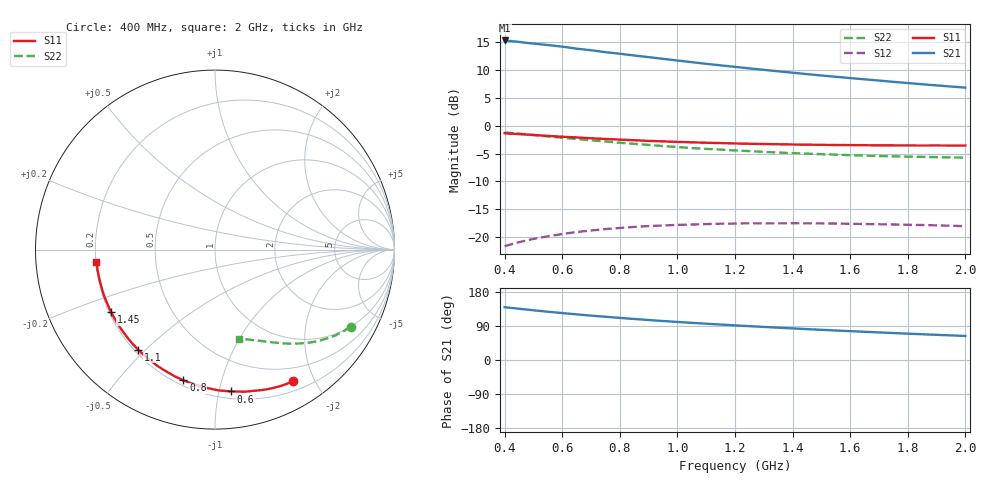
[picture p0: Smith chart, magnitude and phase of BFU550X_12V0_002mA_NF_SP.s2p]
! Filename:  P:\Prog\Test\Noise\ATS_data\Testdata_Net\BFU550X no attenuator noise\BFU550X_APG2013_44_C05_12p0V_002mA_NF_CM01_D.sf
! Date/Time: Fri 26/Jul/2013 14:37:13
! BFU550X_APG2013_44_C05_12p0V_1to10mA_NF_CM01_Bias2_R.sf
! Noise Parameter Data File
! BFU550X_APG2013_44_C05_12p0V_1to10mA_NF_CM01
! Date/time: Thu Jul 25 09:36:35 2013
! VAR V_out= 12.001000
! VAR I_out= 1.995000
! VAR V_in= 0.785500
! VAR I_in= 0.017300
! Device data file deembeded for feedlines and parallel
! Original file: \BFU550X no attenuator noise\BFU550X_APG2013_44_C05_12p0V_002mA_NF_CM01_R.sf
! Feed-files: PR005V01_100713_Feed1.s2p, PR005V01_100713_Feed2.s2p
! Parallel-file: PR005V01_100713_Par.s2p
# MHz S MA R 50
!  Freq-MHz  S11-mag  S11-arg  S21-mag  S21-arg  S12-mag  S12-arg  S22-mag  S22-arg
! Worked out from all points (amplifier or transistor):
!   37 points, 400 MHz to 2 GHz, reference 50 ohm
!   highest |S21| = 15.3 dB at 400 MHz (marker M1)
!   |S21| within 3 dB of that: start of sweep to 902 MHz
!   unconditionally stable (mu >= 1): nowhere
!   at 500 MHz: K = 0.16, MSG = 17.5 dB, |S12| = -20.3 dB
!   at 1.1 GHz: K = 0.33, MSG = 14.4 dB, |S12| = -17.6 dB
!   at 2 GHz: K = 0.62, MSG = 12.4 dB, |S12| = -18.0 dB
!   lowest NFmin = 0.58 dB at 433 MHz
!   S11 on the Smith chart (normalised r, x): 400 MHz: 0.31, -1.71; 600 MHz: 0.25, -1.09; 800 MHz: 0.23, -0.76; 1.1 GHz: 0.22, -0.47; 1.45 GHz: 0.21, -0.27; 2 GHz: 0.20, -0.05
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400  0.8546 -59.3  5.791 139.4  0.08331 55.5  0.8707 -29.8
440  0.8428 -64.5  5.663 136.1  0.08909 52.9  0.8521 -32.0
480  0.8312 -69.3  5.494 132.9  0.09423 50.2  0.8319 -34.2
500  0.824 -71.9  5.434 131.3  0.09676 48.9  0.8252 -35.4
550  0.8095 -77.9  5.268 127.4  0.102 45.9  0.8006 -38.0
600  0.7953 -83.5  5.098 123.8  0.107 43.1  0.7794 -40.3
650  0.7842 -88.8  4.889 120.5  0.1116 40.5  0.7599 -42.4
700  0.7706 -94.0  4.735 117.1  0.115 38.1  0.7388 -44.5
750  0.76 -98.7  4.548 114.1  0.1186 35.9  0.7213 -46.2
800  0.7495 -103.5  4.403 111.1  0.1213 33.7  0.7027 -48.1
850  0.7401 -108.0  4.246 108.2  0.1239 31.7  0.687 -49.7
950  0.7232 -116.4  3.966 102.9  0.1276 28.0  0.656 -52.9
1050  0.709 -124.0  3.702 98.0  0.1301 24.8  0.63 -55.6
1100  0.7028 -127.5  3.577 95.7  0.1313 23.3  0.619 -56.8
1200  0.6926 -134.3  3.36 91.3  0.1328 20.6  0.5992 -59.3
1350  0.6814 -143.4  3.065 85.3  0.1335 17.1  0.5741 -62.6
1450  0.6754 -149.0  2.893 81.5  0.1335 15.0  0.5612 -64.7
1500  0.6729 -151.7  2.812 79.6  0.1332 14.0  0.5553 -65.7
1600  0.6696 -156.8  2.667 76.1  0.1321 12.3  0.5441 -67.7
1750  0.6652 -163.7  2.467 71.1  0.1303 10.2  0.5312 -70.5
1850  0.6639 -168.1  2.348 67.9  0.1289 8.9  0.5256 -72.2
2000  0.6638 -174.2  2.189 63.4  0.1259 7.6  0.5168 -74.9
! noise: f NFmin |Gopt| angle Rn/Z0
400  0.6228  0.4676  29.25  0.1969
460  0.5856  0.4632  39.16  0.1682
600  0.6954  0.4604  45.37  0.2009
800  0.7202  0.453  65.18  0.1639
1000  0.7683  0.4481  79.83  0.1547
1200  0.85  0.4664  95.58  0.1323
1400  0.9364  0.4631  107.9  0.1311
1600  0.7926  0.4878  122.6  0.0946
1800  0.9317  0.4996  138.1  0.0701
2000  1.012  0.5298  149.8  0.0606
